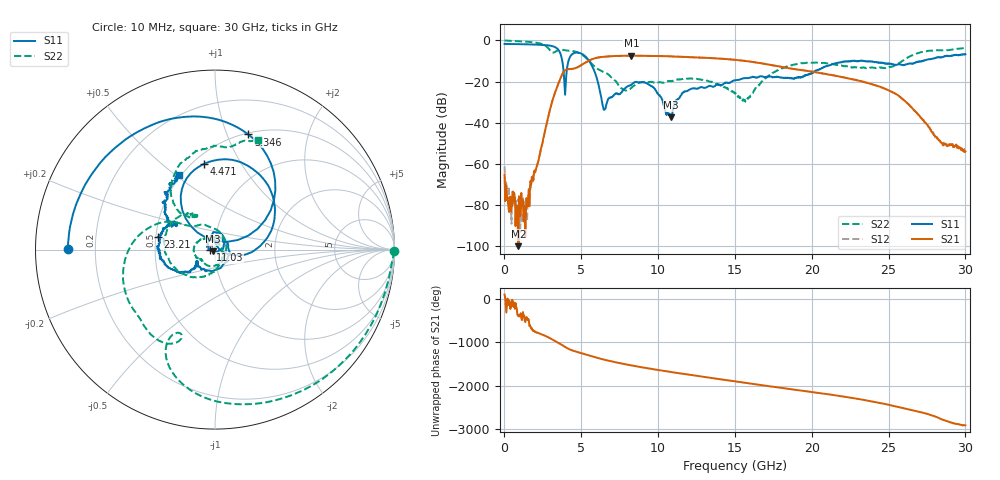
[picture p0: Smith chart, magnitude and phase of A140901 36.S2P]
!  2-Port S-parameters saved by WinCal
! VAR MeasName=S-Parameters (CALIBRATED_DATA) read from VNA (N5244A)
! VAR MeasDate=11/3/2014 9:33:24 AM
! VAR NAME=A140901 36
! VAR FILENAME=A140901 36.S2P
! VAR DATE=11/3/2014 9:33:24 AM
! VAR PHYS_PORTS=1,2
# Hz S RI R 50
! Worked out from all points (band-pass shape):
!   801 points, 10 MHz to 30 GHz, reference 50 ohm
!   highest |S21| = -7.40 dB at 8.257 GHz (marker M1); lowest = -99.9 dB at 909.7 MHz (marker M2)
!   |S21| within 3 dB of the highest: 5.349 GHz to 16.09 GHz (10.75 GHz wide, 100 % of centre)
!   lowest |S11| = -37.4 dB at 10.84 GHz (marker M3), VSWR 1.03, Z = 49 - j0.929 ohm
!   |S11| at or under -10 dB: 3.763 GHz to 4.166 GHz (403.6 MHz wide, 10.2 % of centre); 5.518 GHz to 22.5 GHz (16.98 GHz wide, 121 % of centre); 23.42 GHz to 27.23 GHz (3.813 GHz wide, 15.1 % of centre)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
!   |S22| runs from -29.7 to 0.0 dB; largest |S21 - S12| = 0.003
!   S11 on the Smith chart (normalised r, x): 10 MHz: 0.10, +0.00; 3.346 GHz: 0.52, +1.19; 4.471 GHz: 0.57, +0.70; 11.03 GHz: 0.95, -0.00; 23.21 GHz: 0.51, +0.08; 30 GHz: 0.49, +0.52
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1e7  -0.8184 0.00296  -7.51e-05 0.000544  0.000801 -0.000338  0.9967 -0.00847
3.099e8  -0.8116 0.1009  5.29e-05 -4.32e-05  9.81e-05 7.02e-05  0.9584 -0.1997
9.097e8  -0.758 0.2903  9.27e-06 -4.13e-06  -5.08e-05 0.000135  0.7991 -0.5279
1.472012e9  -0.6613 0.455  2.99e-05 -0.000105  1.16e-05 3.94e-05  0.5409 -0.7569
3.346388e9  0.1854 0.6417  -0.00758 0.0608  -0.00756 0.0606  -0.1947 -0.5039
3.946188e9  0.00513 0.0478  0.1664 -0.0891  0.1664 -0.0885  -0.4029 -0.4113
4.471012e9  -0.0628 0.477  -0.0839 -0.1873  -0.0828 -0.1867  -0.5028 -0.2243
5.033325e9  0.2818 0.3782  -0.2539 -0.0266  -0.2537 -0.0274  -0.452 0.0464
5.820562e9  0.1907 -0.0193  -0.084 0.353  -0.0852 0.3526  -0.19 0.1444
6.495338e9  0.0177 0.0106  0.3096 0.2544  0.3094 0.255  -0.099 0.1343
8.25725e9  -0.0179 0.0822  -0.0136 -0.4262  -0.0135 -0.4248  0.0383 -0.0583
1.001916e10  0.0468 0.0134  -0.3968 0.1312  -0.3962 0.13  -0.0757 -0.0603
1.084389e10  -0.00965 -0.00947  -0.178 0.3683  -0.1786 0.3673  -0.0895 -0.0517
1.103132e10  -0.0265 -0.00109  -0.1109 0.3914  -0.1116 0.3911  -0.0961 -0.0465
1.298068e10  0.0422 0.0572  0.3785 0.0305  0.3786 0.0315  -0.1022 0.0388
1.5005e10  0.0289 -0.1026  -0.052 -0.3332  -0.052 -0.3339  -0.000377 0.0512
1.571726e10  -0.0194 -0.1198  -0.2239 -0.2218  -0.2241 -0.2225  0.0355 0.0066
1.777908e10  -0.1061 -0.0765  -0.1279 0.1989  -0.1292 0.199  -0.1079 -0.1547
2.002832e10  -0.1221 -0.1054  0.1672 0.0477  0.1677 0.0485  -0.2728 0.0855
2.321476e10  -0.318 0.0705  -0.0927 -0.0429  -0.0935 -0.0428  -0.1048 0.1878
2.501416e10  -0.2211 0.1523  0.00835 0.0605  0.00809 0.0607  -0.1276 0.1843
3e10  -0.1979 0.4155  0.00174 -0.00104  0.00169 -0.000828  0.2412 0.6127
